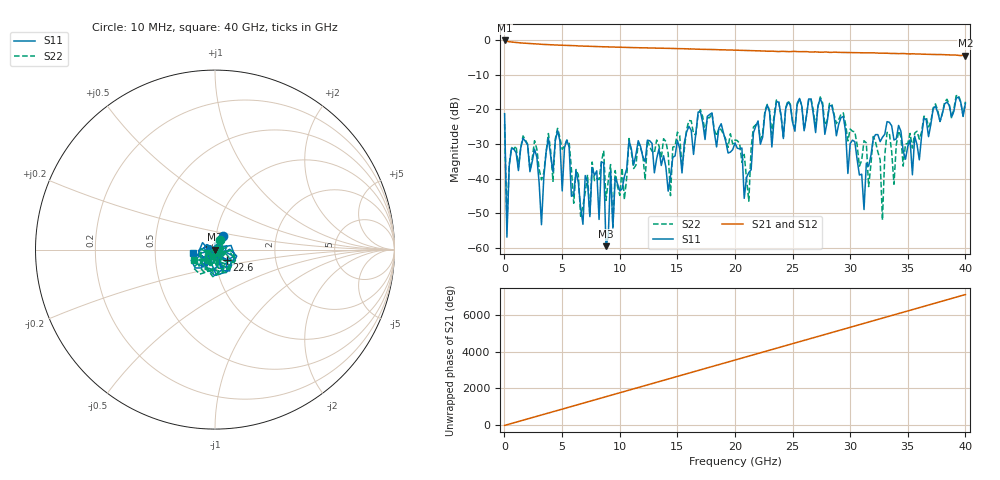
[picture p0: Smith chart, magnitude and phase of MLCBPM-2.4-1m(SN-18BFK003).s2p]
!Keysight Technologies,N5225A,MY51451228,A.10.40.14
!Date: Friday, November 20, 2020 11:44:18
!Correction: S11(Full 2 Port(1,2))
!S21(Full 2 Port(1,2))
!S12(Full 2 Port(1,2))
!S22(Full 2 Port(1,2))
!S2P File: Measurements: S11, S21, S12, S22:
# Hz S  dB  R 50
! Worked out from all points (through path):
!   201 points, 10 MHz to 40 GHz, reference 50 ohm
!   highest |S21| = -0.07 dB at 10 MHz (marker M1); lowest = -4.4 dB at 40 GHz (marker M2)
!   lowest |S11| = -59.5 dB at 8.808 GHz (marker M3), VSWR 1.00, Z = 50 - j0.0963 ohm
!   |S11| at or under -10 dB: start of sweep to end of sweep
!   |S22| runs from -54.0 to -15.9 dB; largest |S21 - S12| = 0.018
!   S11 on the Smith chart (normalised r, x): 10 MHz: 1.08, +0.16; 22.6 GHz: 1.13, -0.14; 40 GHz: 0.78, -0.03
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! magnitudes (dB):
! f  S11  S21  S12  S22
! 10 MHz  -21.2  -0.1  -0.2  -24.2
! 209.9 MHz  -56.9  -0.3  -0.3  -53.3
! 609.9 MHz  -31.2  -0.5  -0.5  -31.0
! 2.609 GHz  -31.5  -1.1  -1.1  -29.0
! 3.209 GHz  -53.3  -1.2  -1.2  -40.3
! 4.609 GHz  -26.1  -1.4  -1.4  -25.5
! 6.808 GHz  -53.2  -1.7  -1.7  -47.8
! 8.608 GHz  -35.4  -1.9  -1.9  -31.9
! 8.808 GHz  -59.5  -1.9  -1.9  -46.3
! 9.208 GHz  -37.7  -1.9  -2.0  -35.9
! 9.408 GHz  -54.3  -2.0  -2.0  -54.0
! 10.81 GHz  -29.0  -2.1  -2.1  -28.4
! 13.41 GHz  -31.4  -2.3  -2.3  -30.5
! 20 GHz  -29.7  -2.9  -2.9  -28.8
! 21.2 GHz  -38.2  -3.0  -3.0  -46.5
! 22.6 GHz  -21.0  -3.1  -3.1  -20.4
! 26.8 GHz  -21.4  -3.4  -3.4  -20.3
! 31.2 GHz  -48.9  -3.6  -3.6  -29.0
! 32.8 GHz  -28.0  -3.7  -3.7  -52.0
! 33.4 GHz  -23.7  -3.8  -3.8  -26.9
! 35.4 GHz  -38.9  -3.9  -3.9  -31.2
! 40 GHz  -18.2  -4.4  -4.4  -17.8
